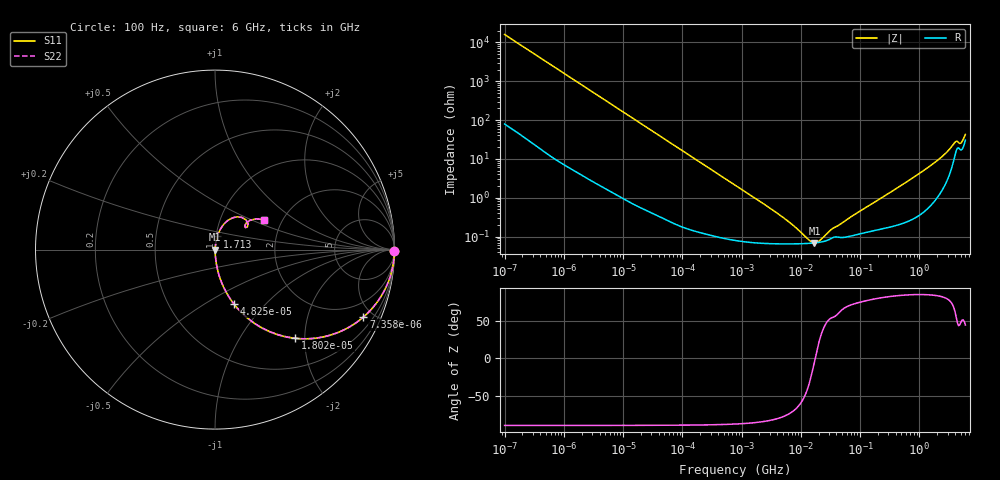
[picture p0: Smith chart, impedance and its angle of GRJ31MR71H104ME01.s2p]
!Murata Part Number: GRJ31MR71H104ME01
!These Parameters are Measured in Series Mode Connection
!Data Generated on Jun 19, 2026
!  o--ll--o
!Port1  Port2
!  o------o
!Operation Temp=25[degC], DC Bias Voltage=0[V]
!Freq. Start=100[Hz] Stop=6[GHz] 401[Steps]
# Hz S RI R 50
!Freq.(Hz) S11(Real) S11(Imag) S21(Real) S21(Imag) S12(Real) S12(Imag) S22(Real) S22(Imag)
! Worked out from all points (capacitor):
!   401 points, 100 Hz to 6 GHz, reference 50 ohm
!   read as one part in series: C = 99.5 nF near 109 Hz
!   lowest |Z| = 68.7 mohm at 17.01 MHz (marker M1)
!   series resonance near 17.5 MHz, so ESL is about 830 pH
!   S11 on the Smith chart (normalised r, x): 100 Hz: open; 7.358 kHz: 1.02, -4.40; 18.02 kHz: 1.01, -1.80; 48.25 kHz: 1.01, -0.68; 1.713 GHz: 1.01, +0.15; 6 GHz: 1.61, +0.60
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100  0.9999 -0.00626  7.01e-05 0.00626  7.01e-05 0.00626  0.9999 -0.00626
627  0.9983 -0.039  0.00169 0.039  0.00169 0.039  0.9983 -0.039
2008  0.9841 -0.1226  0.0159 0.1226  0.0159 0.1226  0.9841 -0.1226
4299  0.9327 -0.248  0.0673 0.248  0.0673 0.248  0.9327 -0.248
7358  0.8272 -0.3753  0.1728 0.3753  0.1728 0.3753  0.8272 -0.3753
12041  0.6435 -0.476  0.3565 0.476  0.3565 0.476  0.6435 -0.476
18016  0.4482 -0.4941  0.5518 0.4941  0.5518 0.4941  0.4482 -0.4941
40335  0.1421 -0.3451  0.8579 0.3451  0.8579 0.3451  0.1421 -0.3451
48246  0.1044 -0.3016  0.8956 0.3016  0.8956 0.3016  0.1044 -0.3016
154540  0.0125 -0.1045  0.9875 0.1045  0.9875 0.1045  0.0125 -0.1045
774597  0.00124 -0.0212  0.9988 0.0212  0.9988 0.0212  0.00124 -0.0212
5079039  0.000654 -0.00299  0.9993 0.00299  0.9993 0.00299  0.000654 -0.00299
1.555665e7  0.000676 -0.000223  0.9993 0.000223  0.9993 0.000223  0.000676 -0.000223
1.701401e7  0.000684 -5.25e-05  0.9993 5.25e-05  0.9993 5.25e-05  0.000684 -5.25e-05
2.035112e7  0.000708 0.000288  0.9993 -0.000288  0.9993 -0.000288  0.000708 0.000288
3.482834e7  0.000941 0.00133  0.9991 -0.00133  0.9991 -0.00133  0.000941 0.00133
3.124326e8  0.0019 0.0131  0.9981 -0.0131  0.9981 -0.0131  0.0019 0.0131
1.712697e9  0.0127 0.0732  0.9873 -0.0732  0.9873 -0.0732  0.0127 0.0732
2.931063e9  0.0463 0.1378  0.9537 -0.1378  0.9537 -0.1378  0.0463 0.1378
3.8344e9  0.1244 0.1824  0.8756 -0.1824  0.8756 -0.1824  0.1244 0.1824
5.016141e9  0.166 0.1338  0.834 -0.1338  0.834 -0.1338  0.166 0.1338
6e9  0.2716 0.1671  0.7284 -0.1671  0.7284 -0.1671  0.2716 0.1671
